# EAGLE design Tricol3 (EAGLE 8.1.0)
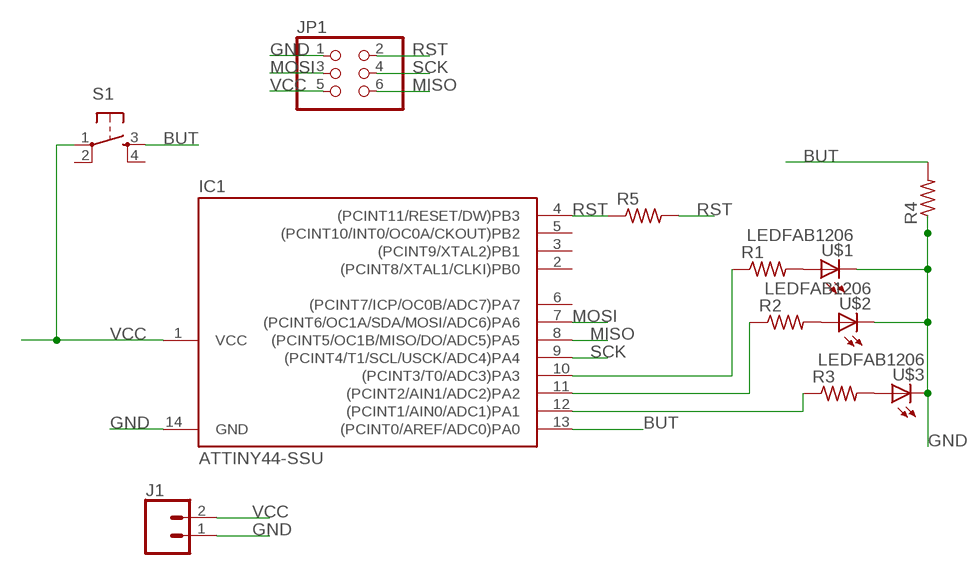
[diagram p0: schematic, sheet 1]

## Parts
IC1  ATTINY44-SSU  [SOIC14]
J1  CONN_02PTH3  [1X02_LONGPADS]
JP1  PINHD-2X3-SMD  [2X03SMD]
R1  RES-US1206FAB  [R1206FAB]
R2  RES-US1206FAB  [R1206FAB]
R3  RES-US1206FAB  [R1206FAB]
R4  RES-US1206FAB  [R1206FAB]
R5  RES-US1206FAB  [R1206FAB]
S1  6MM_SWITCH6MM_SWITCH  [6MM_SWITCH]
U$1  LEDFAB1206  [LED1206FAB]
U$2  LEDFAB1206  [LED1206FAB]
U$3  LEDFAB1206  [LED1206FAB]

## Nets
BUT: IC1.13((PCINT0/AREF/ADC0)PA0) R4.2 S1.3(S)
GND: IC1.14(GND) J1.1 JP1.1 R4.1 U$1.2(C) U$2.2(C) U$3.2(C)
MISO: IC1.8((PCINT5/OC1B/MISO/DO/ADC5)PA5) JP1.6
MOSI: IC1.7((PCINT6/OC1A/SDA/MOSI/ADC6)PA6) JP1.3
N$1: IC1.10((PCINT3/T0/ADC3)PA3) R1.1
N$2: IC1.11((PCINT2/AIN1/ADC2)PA2) R2.1
N$3: IC1.12((PCINT1/AIN0/ADC1)PA1) R3.1
N$4: R1.2 U$1.1(A)
N$5: R2.2 U$2.1(A)
N$6: R3.2 U$3.1(A)
RST: IC1.4((PCINT11/RESET/DW)PB3) JP1.2 R5.1 R5.2
SCK: IC1.9((PCINT4/T1/SCL/USCK/ADC4)PA4) JP1.4
VCC: IC1.1(VCC) J1.2 JP1.5 S1.1(P)
Unconnected: IC1.2((PCINT8/XTAL1/CLKI)PB0) IC1.3((PCINT9/XTAL2)PB1) IC1.5((PCINT10/INT0/OC0A/CKOUT)PB2) IC1.6((PCINT7/ICP/OC0B/ADC7)PA7) S1.2(P1) S1.4(S1)

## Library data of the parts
IC1 = fab:ATTINY44
J1 = SparkFun-Connectors:CONN_02: Multi connection point. Often used as Generic Header-pin footprint for 0.1 inch spaced/style header connections
JP1 = fab:PINHD-2X3-SMD: PIN HEADER
R1-R5 = fab:RES-US: Resistor (US Symbol)
S1 = fab:6MM_SWITCH: OMRON SWITCH
U$1-U$3 = fab:LED: LED

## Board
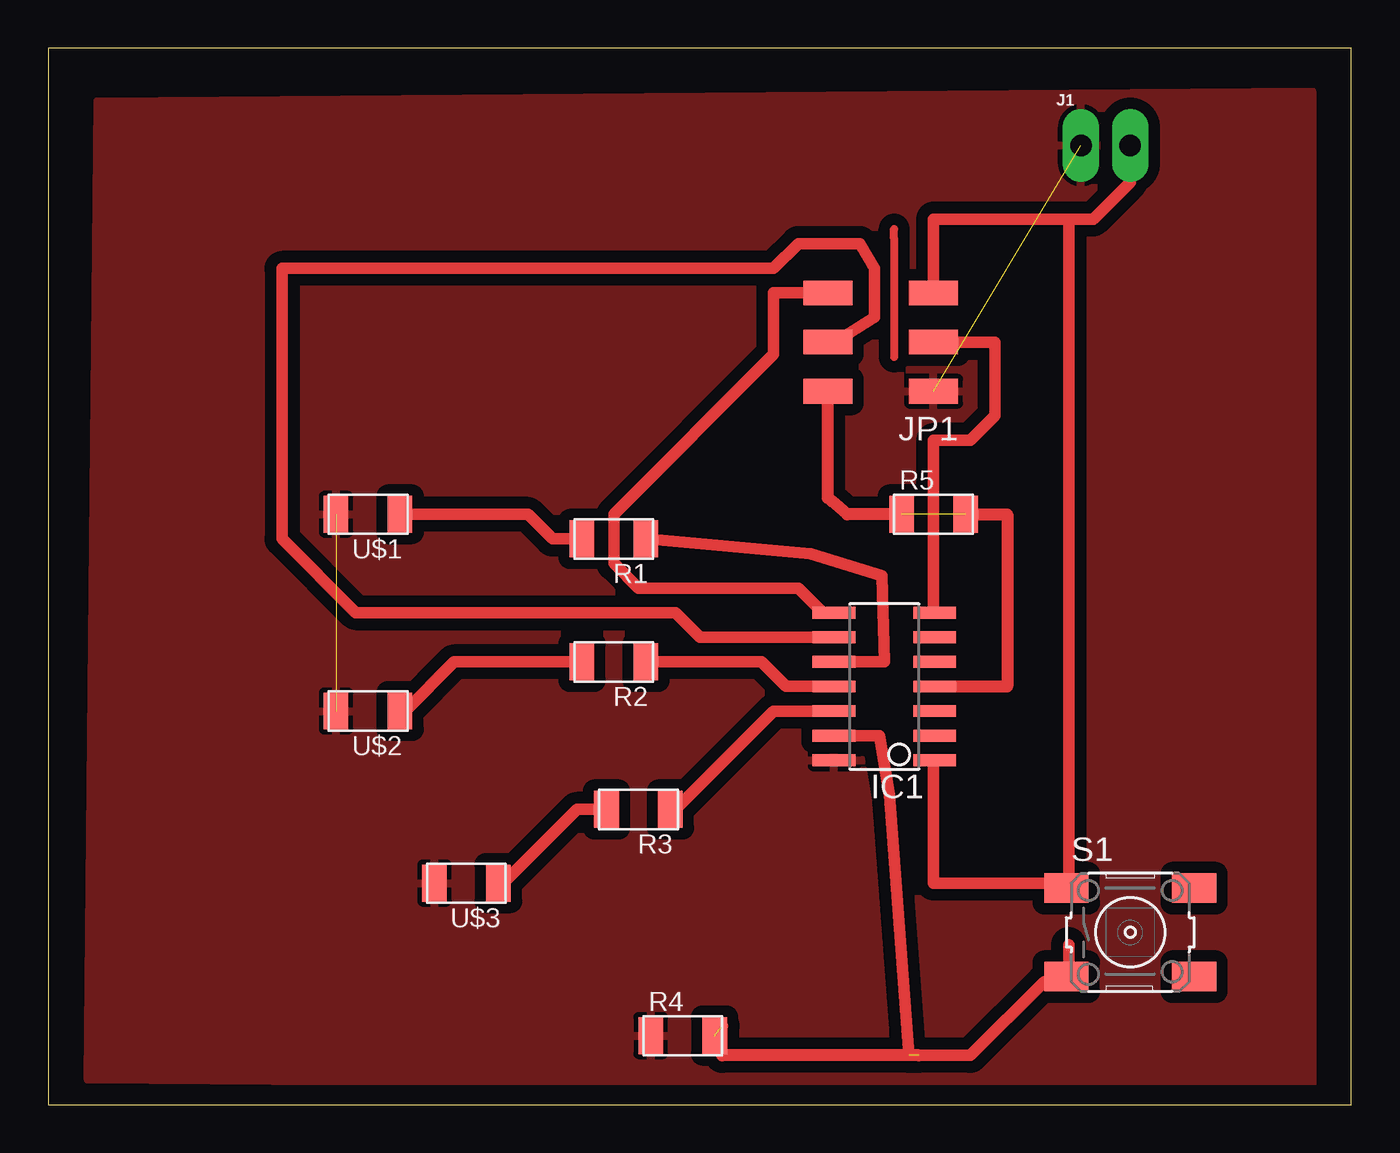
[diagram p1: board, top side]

Size 67.29 x 54.53 mm. Coordinates in mm from the lower left corner, seen from the top.
Outline: 0,0 67.29,0 67.29,54.53 0,54.53 0,0
Copper layers (1*16): Top 0.4mm / dielectric 0.4mm / Bottom 0.4mm
Design rules "default *": minimum track width 0.6mm, minimum drill 24mil, track to track 0.6mm, track to pad 0.6mm, pad to pad 0.6mm, via to via 8mil, smd to smd 8mil, copper to edge 40mil, drill to drill 8mil, minimum pad ring 10mil, minimum via ring 8mil, stop-mask expansion 4mil, vias tented up to drill 0mil, thermal gap 10mil

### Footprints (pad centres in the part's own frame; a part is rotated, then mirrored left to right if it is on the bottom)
SOIC14 = smd 0.61 x 2.21: 1 -3.81,-2.603; 2 -2.54,-2.603; 3 -1.27,-2.603; 4 0,-2.603; 5 1.27,-2.603; 6 2.54,-2.603; 7 3.81,-2.603; 8 3.81,2.603; 9 2.54,2.603; 10 1.27,2.603; 11 0,2.603; 12 -1.27,2.603; 13 -2.54,2.603; 14 -3.81,2.603
1X02_LONGPADS = drill 1.118 pad 1.88 long: 1 0,0; 2 2.54,0
2X03SMD = smd 2.54 x 1.27: 1 -2.54,2.54; 2 2.92,2.54; 3 -2.54,0; 4 2.92,0; 5 -2.54,-2.54; 6 2.92,-2.54
R1206FAB = smd 1.27 x 1.905: 1 -1.651,0; 2 1.651,0
6MM_SWITCH = smd 2.286 x 1.524: 1 -3.302,2.286; 2 3.302,2.286; 3 -3.302,-2.286; 4 3.302,-2.286
LED1206FAB = smd 1.27 x 1.905: 1 -1.651,0; 2 1.651,0

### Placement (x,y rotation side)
IC1  43.18,21.59 90 top
J1  53.34,49.53 0 top
JP1  43.18,39.37 180 top
R1  29.21,29.21 180 top
R2  29.21,22.86 180 top
R3  30.48,15.24 180 top
R4  32.77,3.56 0 top
R5  45.72,30.48 0 top
S1  55.88,8.89 0 top
U$1  16.51,30.48 180 top
U$2  16.51,20.32 180 top
U$3  21.59,11.43 180 top

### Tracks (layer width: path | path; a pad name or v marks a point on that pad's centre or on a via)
BUT  (2 unrouted)
  Top 0.6: 52.71,6.35 S1.3 | IC1.13 42.93,19.05 43.43,16 44.45,2.54 47.62,2.54 51.44,6.35 52.07,6.35 S1.3 | 52.71,8.25 52.71,6.98 S1.3
  Top 0.61: 44.96,2.54 34.8,2.54 34.8,4.06
GND  (2 unrouted)
  pour Top: 2.54,51.82 65.28,52.32 65.28,0.76 2.03,1.27
MISO
  Top 0.6: JP1.6 37.47,41.91 37.47,38.73 29.21,30.48 29.21,27.94 30.48,26.67 38.73,26.67 40.01,25.4 IC1.8
MOSI
  Top 0.6: JP1.3 48.9,39.37 48.9,35.56 47.62,34.29 45.72,34.29 45.72,25.4 IC1.7
N$1
  Top 0.6: R1.1 39.37,28.45 43.05,27.31 43.18,22.86 IC1.10
N$2
  Top 0.6: R2.1 36.83,22.86 38.1,21.59 IC1.11
N$3
  Top 0.6: IC1.12 37.47,20.32 32.38,15.24 R3.1
N$4
  Top 0.6: U$1.1 24.77,30.48 26.04,29.21 R1.2
N$5
  Top 0.6: R2.2 20.95,22.86 18.41,20.32 U$2.1
N$6
  Top 0.6: R3.2 27.3,15.24 23.49,11.43 U$3.1
N$7
  Top 0.406: 43.69,38.61 43.69,44.7 43.69,45.21
RST  (1 unrouted)
  Top 0.6: JP1.2 40.01,36.83
  Top 0.61: IC1.4 49.53,21.59 49.53,30.48 R5.2 | JP1.2 40.26,31.32 40.49,31.15 41.27,30.48 R5.1
SCK
  Top 0.6: IC1.9 33.66,24.13 32.38,25.4 15.88,25.4 12.07,29.21 12.07,43.18 37.47,43.18 38.73,44.45 41.91,44.45 42.67,43.18 42.67,40.64 40.64,39.37 JP1.4
VCC
  Top 0.6: IC1.1 45.72,17.78 45.72,11.43 52.07,11.43 S1.1 52.71,11.43 52.71,45.72 | JP1.5 45.72,45.72 52.71,45.72 | 52.71,45.72 53.98,45.72 55.88,47.62 J1.2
